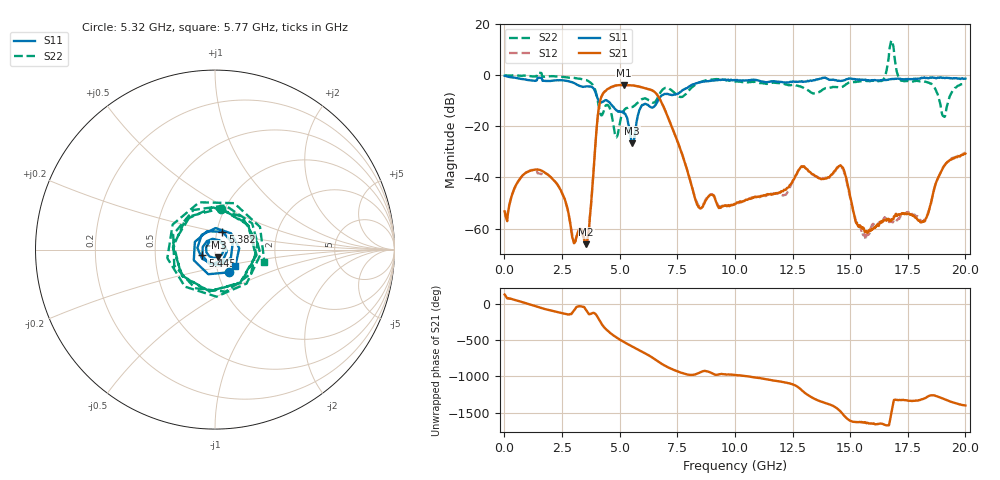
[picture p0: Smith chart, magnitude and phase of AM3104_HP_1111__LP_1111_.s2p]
!Created with skrf (http://scikit-rf.org).
# Hz S RI R 50.0
!freq ReS11 ImS11 ReS21 ImS21 ReS12 ImS12 ReS22 ImS22
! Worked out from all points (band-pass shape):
!   1601 points, 10 MHz to 20 GHz, reference 50 ohm
!   highest |S21| = -3.83 dB at 5.182 GHz (marker M1); lowest = -66.1 dB at 3.546 GHz (marker M2)
!   |S21| within 3 dB of the highest: 4.307 GHz to 6.552 GHz (2.245 GHz wide, 41.3 % of centre)
!   lowest |S11| = -26.6 dB at 5.545 GHz (marker M3), VSWR 1.10, Z = 51.7 - j4.45 ohm
!   |S11| at or under -10 dB: 4.093 GHz to 4.342 GHz (249.6 MHz wide, 5.92 % of centre); 4.469 GHz to 6.658 GHz (2.189 GHz wide, 39.3 % of centre)
!   |S22| runs from -24.3 to 13.6 dB; largest |S21 - S12| = 0.078
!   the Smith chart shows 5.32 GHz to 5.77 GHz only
!   S11 on the Smith chart (normalised r, x): 5.32 GHz: 1.13, -0.29; 5.382 GHz: 1.06, +0.21; 5.445 GHz: 0.87, -0.06; 5.77 GHz: 1.23, -0.23
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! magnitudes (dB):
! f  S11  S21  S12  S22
! 10 MHz  -0.2  -53.3  -54.4  0.0
! 1.509 GHz  -1.0  -37.0  -38.5  0.9
! 3.346 GHz  -4.4  -60.5  -60.2  -1.5
! 3.546 GHz  -4.4  -66.1  -66.9  -1.9
! 4.17 GHz  -10.7  -9.5  -9.6  -15.2
! 4.858 GHz  -13.7  -4.0  -4.0  -24.3
! 5.182 GHz  -14.8  -3.8  -3.9  -13.9
! 5.32 GHz  -16.5  -3.9  -3.9  -12.8
! 5.382 GHz  -19.4  -3.9  -3.9  -12.5
! 5.445 GHz  -22.2  -3.9  -3.9  -12.6
! 5.545 GHz  -26.6  -4.0  -4.0  -12.4
! 5.77 GHz  -16.8  -4.3  -4.3  -11.0
! 6.682 GHz  -9.6  -8.3  -8.4  -8.2
! 8.418 GHz  -2.9  -51.6  -50.9  -2.9
! 10.01 GHz  -2.0  -50.4  -50.4  -2.5
! 13.34 GHz  -2.2  -38.6  -38.7  -6.9
! 14.63 GHz  -2.2  -35.7  -36.0  -4.7
! 15.6 GHz  -1.9  -60.2  -62.5  -2.3
! 16.68 GHz  -1.7  -56.7  -57.0  7.3
! 18.2 GHz  -0.9  -57.2  -57.0  -2.4
! 19.05 GHz  -1.0  -35.8  -35.7  -16.0
! 20 GHz  -1.3  -30.7  -30.3  -3.0
